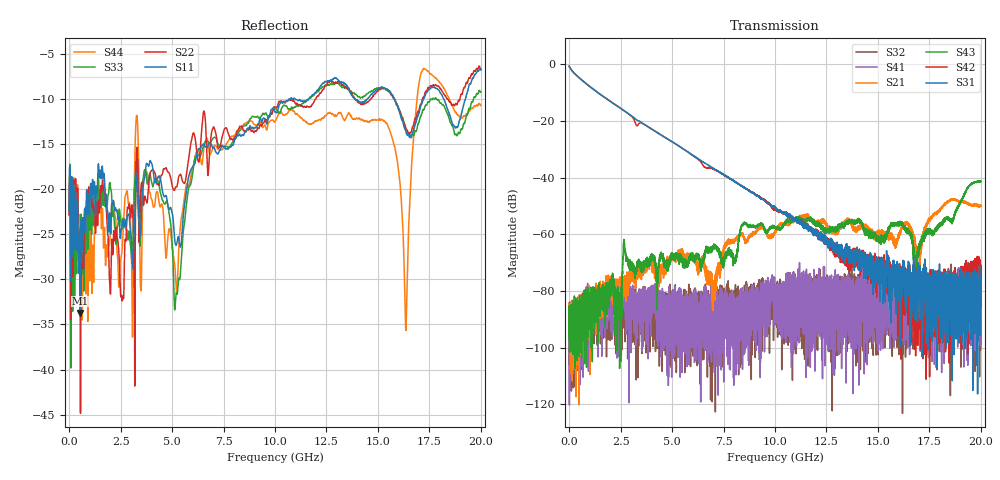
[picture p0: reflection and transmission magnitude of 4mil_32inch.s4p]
!Agilent Technologies,N5230A,US43500443,A.06.04.32
!Agilent N5230A: A.06.04.32
!Date: Wednesday, December 12, 2012 16:55:36
!Correction: S11(Full 4 Port(1,2,3,4)) S12(Full 4 Port(1,2,3,4)) S13(Full 4 Port(1,2,3,4)) S14(Full 4 Port(1,2,3,4)) S21(Full 4 Port(1,2,3,4)) S22(Full 4 Port(1,2,3,4)) S23(Full 4 Port(1,2,3,4)) S24(Full 4 Port(1,2,3,4)) S31(Full 4 Port(1,2,3,4)) S32(Full 4 Port(1,2,3,4)) S33(Full 4 Port(1,2,3,4)) S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
!S4P File: Measurements: <S11,S12,S13,S14>, <S21,S22,S23,S24>, <S31,S32,S33,S34>, <S41,S42,S43,S44>:
# Hz S  dB  R 50
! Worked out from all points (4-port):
!   10000 points, 1 MHz to 20 GHz, reference 50 ohm
!   strongest paths, dB at 1 MHz, 5.001 GHz, 10 GHz, 15 GHz, 20 GHz:
!     S31: -0.7, -27.3, -50.4, -71.0, -82.7
!     S42: -0.7, -27.3, -51.0, -72.0, -76.0
!     S43: -94.3, -66.6, -57.4, -61.7, -41.3
!     S21: -95.4, -67.7, -59.6, -60.2, -50.0
!     S41: -87.6, -85.4, -85.5, -81.7, -82.2
!     S32: -84.4, -84.1, -85.3, -87.9, -80.8
!   lowest |S11| = -33.7 dB at 531 MHz (marker M1), VSWR 1.04, Z = 50.2 - j2.05 ohm
!   |S11| at or under -10 dB: start of sweep to 10.67 GHz; 15.81 GHz to 17.21 GHz (1.399 GHz wide, 8.47 % of centre); 18.21 GHz to 19.24 GHz (1.038 GHz wide, 5.55 % of centre)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
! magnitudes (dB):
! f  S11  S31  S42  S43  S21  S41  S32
! 1 MHz  -22.4  -0.7  -0.7  -94.3  -95.4  -87.6  -84.4
! 531 MHz  -33.7  -5.0  -5.0  -87.9  -90.7  -90.2  -84.4
! 8.513 GHz  -13.7  -43.5  -43.5  -56.2  -61.6  -87.8  -84.4
! 15.15 GHz  -8.7  -70.3  -74.4  -61.2  -59.1  -76.7  -92.2
! 16.35 GHz  -13.5  -86.8  -73.2  -57.6  -55.8  -82.3  -80.7
! 16.84 GHz  -12.6  -78.9  -83.0  -72.4  -65.7  -75.2  -82.8
! 20 GHz  -6.7  -82.7  -76.0  -41.3  -50.0  -82.2  -80.8
